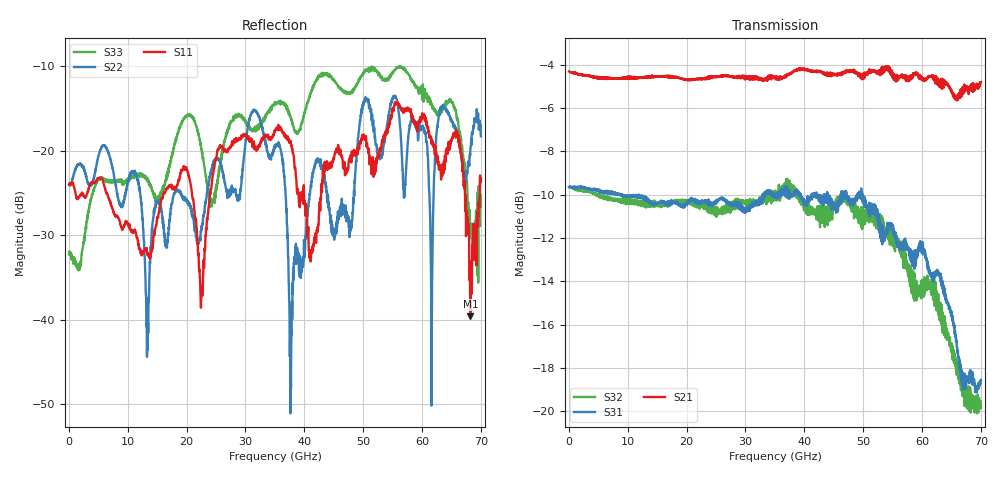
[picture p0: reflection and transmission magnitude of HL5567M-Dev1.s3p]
! 2/10/2020 1:47:33 PM
! H:\PROTOTYPE_DATA\HL9467M\LA01A.S3P
! CHANNEL.1
! TR.MEASUREMENT
! CORRECTED.DATA
# GHZ S RI R 50.0
! FREQ.GHZ  S11RE  S11IM  S12RE  S12IM  S13RE  S13IM
!  S21RE  S21IM  S22RE  S22IM  S23RE  S23IM
!  S31RE  S31IM  S32RE  S32IM  S33RE  S33IM
!; PortSelection: Port_123
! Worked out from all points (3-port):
!   2000 points, 35 MHz to 70 GHz, reference 50 ohm
!   strongest paths, dB at 35 MHz, 17.54 GHz, 35.03 GHz, 52.53 GHz, 70 GHz:
!     S21: -4.3, -4.6, -4.6, -4.4, -4.8
!     S31: -9.6, -10.3, -10.0, -11.2, -18.5
!     S32: -9.6, -10.3, -10.2, -11.1, -19.8
!   lowest |S11| = -39.6 dB at 68.22 GHz (marker M1), VSWR 1.02, Z = 50.6 - j0.896 ohm
!   |S11| at or under -10 dB: start of sweep to end of sweep
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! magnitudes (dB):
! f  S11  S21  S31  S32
! 35 MHz  -24.1  -4.3  -9.6  -9.6
! 11.2 GHz  -29.4  -4.6  -10.0  -10.2
! 13.34 GHz  -32.3  -4.5  -10.3  -10.5
! 35.03 GHz  -17.7  -4.6  -10.0  -10.2
! 37.7 GHz  -19.0  -4.4  -10.1  -9.8
! 50.37 GHz  -18.5  -4.4  -10.2  -10.9
! 61.6 GHz  -19.2  -4.5  -13.8  -14.0
! 63.17 GHz  -22.2  -5.0  -13.9  -15.9
! 68.22 GHz  -39.6  -5.0  -18.5  -19.3
! 70 GHz  -23.3  -4.8  -18.5  -19.8
